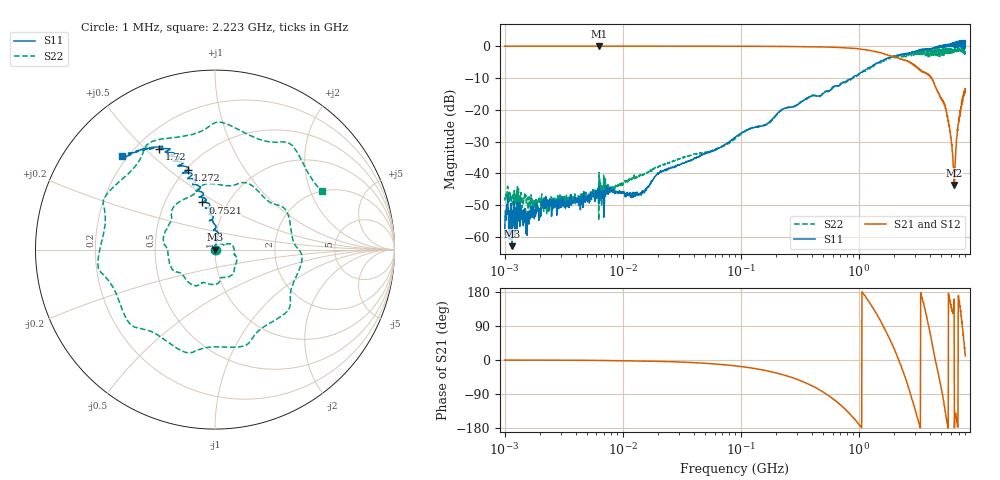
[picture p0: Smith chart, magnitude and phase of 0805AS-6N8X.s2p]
!s-Parameter Generated by FASTRON Sdn. Bhd.
!FASTRON P/N : 0805AS-6N8X
!Keysight Technologies: E5071C_MY46733604_B.14.02
!Date: Mon Jun 15 12:47:30 2026
!Version  :Rev01  Mon Jun 15 12:47:30 2026
!Data & Calibration Information:
!Freq  S11:SOLT2(ON)  S21:SOLT2(ON)  S12:SOLT2(ON)  S22:SOLT2(ON)
!PortZ  Port1:50+j0  Port2:50+j0
!When reading reference impedance value at option line is always used.
! Remarks : This data is being provided solely for informational purposes.
# Hz S dB R 50
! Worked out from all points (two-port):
!   1601 points, 1 MHz to 8 GHz, reference 50 ohm
!   highest |S21| = 0.00 dB at 6.301 MHz (marker M1); lowest = -43.6 dB at 6.419 GHz (marker M2)
!   |S21| within 3 dB of the highest: start of sweep to 1.837 GHz
!   lowest |S11| = -62.8 dB at 1.152 MHz (marker M3), VSWR 1.00, Z = 50.1 + j0.00927 ohm
!   |S11| at or under -10 dB: start of sweep to 895.6 MHz
!   |S22| runs from -54.7 to -0.7 dB; largest |S21 - S12| = 0.016
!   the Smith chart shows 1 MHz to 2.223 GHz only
!   S11 on the Smith chart (normalised r, x): 1 MHz: 1.00, +0.00; 752.1 MHz: 0.76, +0.43; 1.272 GHz: 0.51, +0.58; 1.72 GHz: 0.29, +0.55; 2.223 GHz: 0.18, +0.40
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1000000  -59.20 11.8  -0.06 -0.2  -0.03 -0.2  -48.50 8.4
1151819  -62.80 7.3  -0.06 -0.2  -0.03 -0.2  -47.50 9.3
4479405  -49.10 34.3  -0.04 -0.8  -0.04 -0.9  -48.30 37.9
6301378  -44.10 43.3  0.00 -1.3  -0.03 -1.1  -39.70 43.0
2.00676e7  -39.90 73.0  -0.05 -3.5  -0.05 -3.5  -37.90 57.1
8.994653e7  -28.60 78.0  -0.07 -15.5  -0.08 -15.5  -29.00 50.6
4.006501e8  -15.60 94.8  -0.26 -67.9  -0.26 -67.9  -15.50 -53.5
7.521334e8  -11.30 105.0  -0.53 -127.0  -0.53 -127.0  -11.60 -177.0
1.272209e9  -6.60 109.0  -1.51 145.0  -1.50 145.0  -6.50 -1.0
1.720333e9  -3.88 119.0  -2.63 72.2  -2.64 72.1  -4.40 -156.0
1.7949e9  -3.69 119.0  -2.95 60.8  -2.94 60.6  -3.78 -178.0
2.222796e9  -2.66 135.0  -3.90 -7.8  -3.91 -7.8  -3.37 28.5
2.545586e9  -2.48 143.0  -4.77 -58.0  -4.78 -58.0  -2.44 -80.7
2.839031e9  -2.05 144.0  -5.81 -106.0  -5.81 -106.0  -1.99 180.0
3.365624e9  -1.26 166.0  -7.56 174.0  -7.52 174.0  -2.27 2.5
3.872345e9  -0.83 -176.0  -8.86 94.9  -8.84 94.5  -3.34 -177.0
4.380627e9  -0.48 -179.0  -12.00 10.3  -12.00 9.6  -2.20 8.2
4.940464e9  0.04 -136.0  -16.40 -65.4  -16.40 -66.0  -3.13 -176.0
5.472309e9  -0.03 -135.0  -19.90 -149.0  -19.80 -148.0  -1.40 6.9
5.995147e9  0.07 -102.0  -28.60 146.0  -28.60 146.0  -0.97 -160.0
6.419251e9  1.15 -63.0  -43.60 161.0  -43.70 161.0  -1.91 64.8
8e9  1.68 -24.3  -13.50 11.0  -13.30 11.7  -3.13 -110.0
